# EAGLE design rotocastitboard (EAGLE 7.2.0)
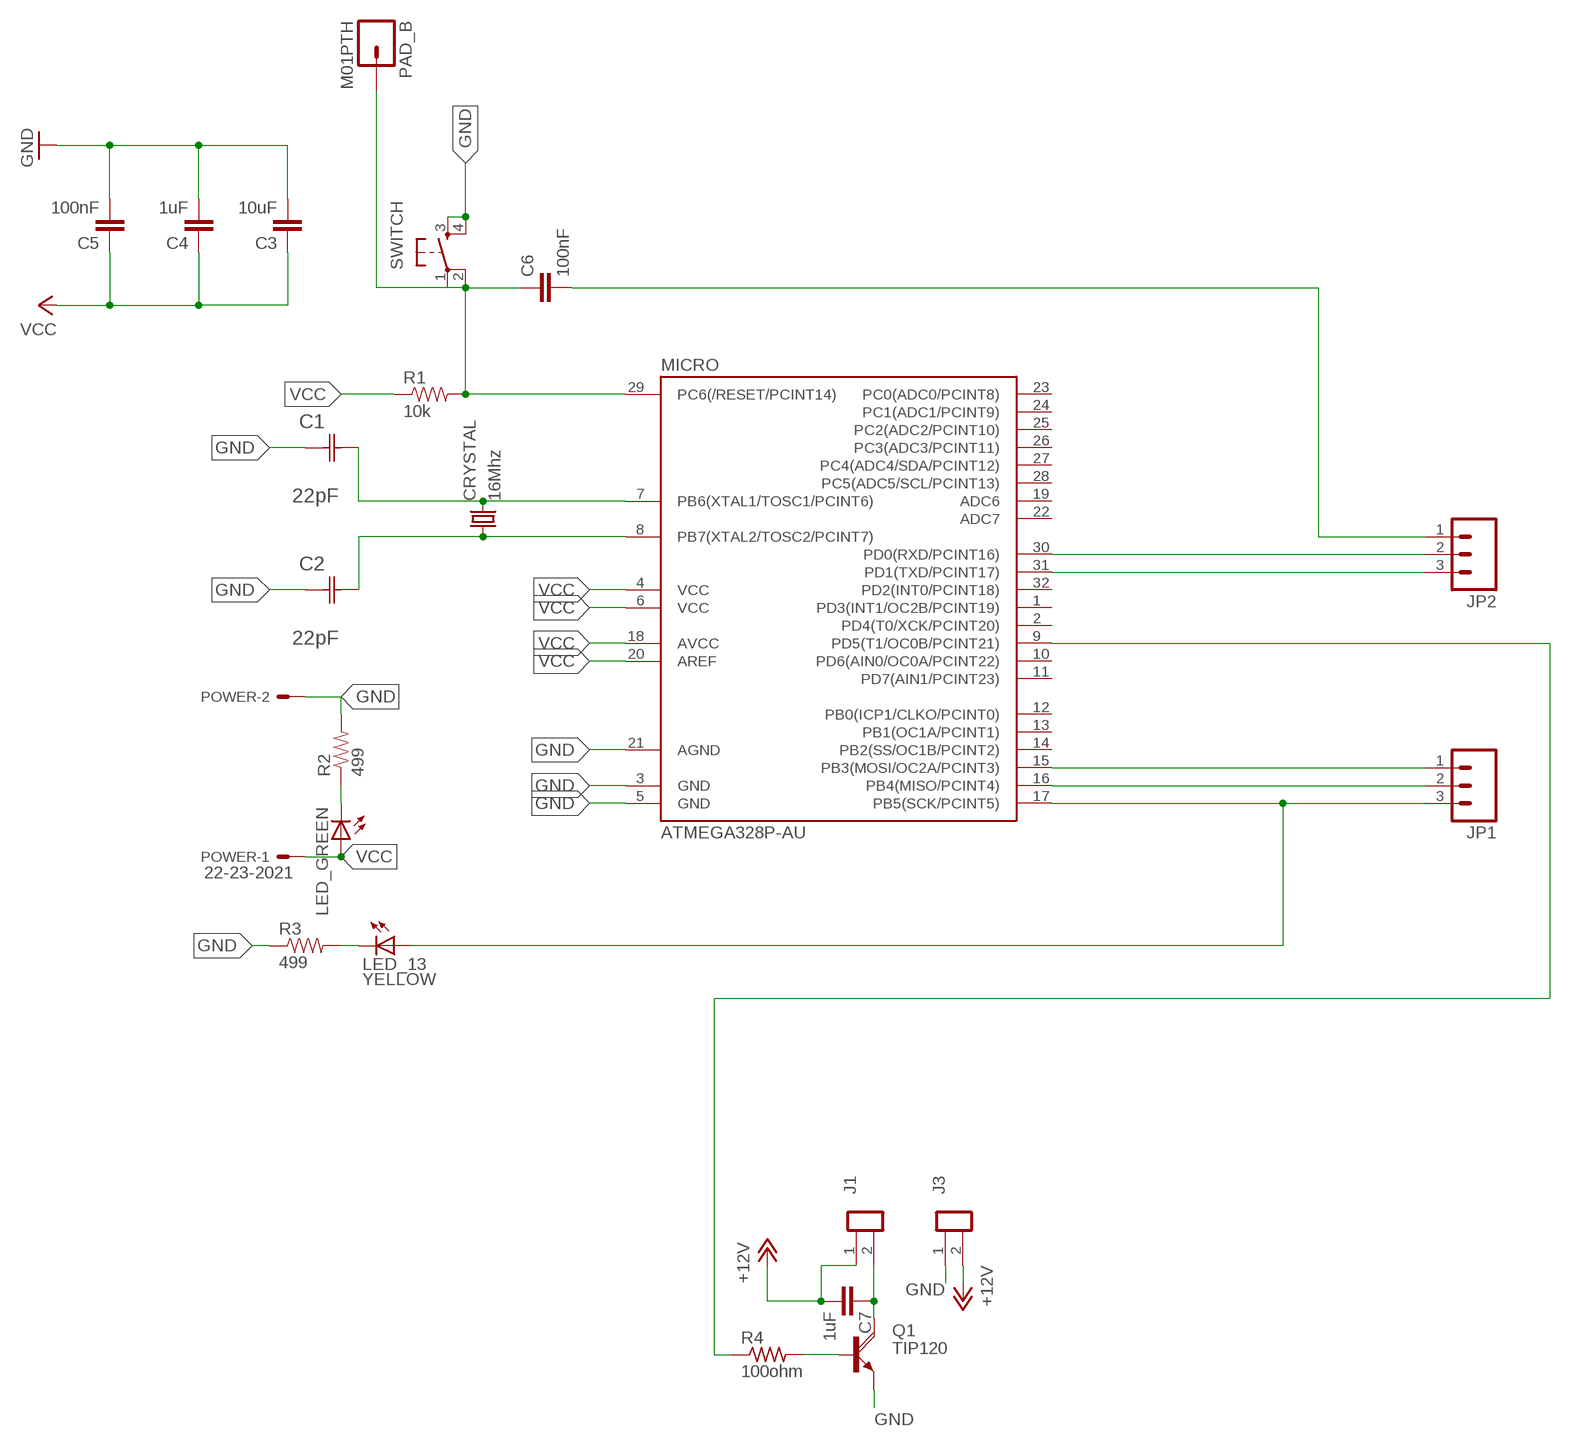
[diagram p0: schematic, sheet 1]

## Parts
C1  22pF  0612ZC225MAT2A  [CAPC3216X178N]
C2  22pF  0612ZC225MAT2A  [CAPC3216X178N]
C3  10uF  CAP1206  [1206]
C4  1uF  CAP1206  [1206]
C5  100nF  CAP1206  [1206]
C6  100nF  CAP1206  [1206]
C7  1uF  CAP1206  [1206]
CRYSTAL  16Mhz  CSM-7X-DU  [CSM-7X-DU]
J1  ED550-2  [ED550-2]
J3  ED550-2  [ED550-2]
JP1  M031X03_NO_SILK  [1X03_NO_SILK]
JP2  M031X03_NO_SILK  [1X03_NO_SILK]
LED_13  YELLOW  LED1206  [1206]
LED_GREEN  LED1206  [1206]
MICRO  ATMEGA328P-AU  ATMEGA48/88/168-AU  [TQFP32-08]
PAD_B  M01PTH  [1X01]
POWER  22-23-2021  [22-23-2021]
Q1  TIP120  [TO220AH]
R1  10k  RESISTOR1206  [1206]
R2  499  RESISTOR1206  [1206]
R3  499  RESISTOR1206  [1206]
R4  100ohm  RESISTOR1206  [1206]
SWITCH  6MM_SWITCH6MM_SWITCH  [6MM_SWITCH]

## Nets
+12V: C7.2 J1.1 J3.2
GND: C1.1(C1) C2.1(C1) C3.2 C4.2 C5.2 J3.1 MICRO.3(GND) MICRO.5(GND) MICRO.21(AGND) POWER.2 Q1.E R2.2 R3.1 SWITCH.3(S) SWITCH.4(S1)
N$1: C6.2 JP2.1
N$2: C1.2(C2) CRYSTAL.2 MICRO.7(PB6(XTAL1/TOSC1/PCINT6))
N$3: Q1.B R4.2
N$4: C7.1 J1.2 Q1.C
N$9: C2.2(C2) CRYSTAL.1 MICRO.8(PB7(XTAL2/TOSC2/PCINT7))
N$10: JP1.1 MICRO.15(PB3(MOSI/OC2A/PCINT3))
N$11: JP1.2 MICRO.16(PB4(MISO/PCINT4))
N$12: JP1.3 LED_13.1(A) MICRO.17(PB5(SCK/PCINT5))
N$20: JP2.2 MICRO.30(PD0(RXD/PCINT16))
N$21: JP2.3 MICRO.31(PD1(TXD/PCINT17))
N$26: LED_GREEN.2(C) R2.1
N$27: LED_13.2(C) R3.2
N$28: C6.1 MICRO.29(PC6(/RESET/PCINT14)) PAD_B.1 R1.2 SWITCH.1(P) SWITCH.2(P1)
N$34: MICRO.9(PD5(T1/OC0B/PCINT21)) R4.1
VCC: C3.1 C4.1 C5.1 LED_GREEN.1(A) MICRO.4(VCC) MICRO.6(VCC) MICRO.18(AVCC) MICRO.20(AREF) POWER.1 R1.1
Unconnected: MICRO.1(PD3(INT1/OC2B/PCINT19)) MICRO.2(PD4(T0/XCK/PCINT20)) MICRO.10(PD6(AIN0/OC0A/PCINT22)) MICRO.11(PD7(AIN1/PCINT23)) MICRO.12(PB0(ICP1/CLKO/PCINT0)) MICRO.13(PB1(OC1A/PCINT1)) MICRO.14(PB2(SS/OC1B/PCINT2)) MICRO.19(ADC6) MICRO.22(ADC7) MICRO.23(PC0(ADC0/PCINT8)) MICRO.24(PC1(ADC1/PCINT9)) MICRO.25(PC2(ADC2/PCINT10)) MICRO.26(PC3(ADC3/PCINT11)) MICRO.27(PC4(ADC4/SDA/PCINT12)) MICRO.28(PC5(ADC5/SCL/PCINT13)) MICRO.32(PD2(INT0/PCINT18))

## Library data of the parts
C1 C2 = AVX_By_element14_Batch_1:0612ZC225MAT2A: Capacitor 1206; MPN: 0612ZC225MAT2A; OC_FARNELL: -; OC_NEWARK: 12N3209; SUPPLIER: AVX; TOLERANCE: ±20%; VALUE: 2.2µF; VOLTAGERATING: 10V
C3-C7 = 01_SparkFun:CAP: Capacitor
CRYSTAL = 01_FAB_Hello:CSM-7X-DU: SMD CRYSTAL; OC_FARNELL: unknown; OC_NEWARK: unknown
J1 J3 = ads:ED550-2
JP1 JP2 = 01_SparkFun:M03: Header 3 Standard 3-pin 0.1" header. Use with straight break away headers (SKU : PRT-00116), right angle break away headers (PRT-00553), swiss pins (PRT-00743), machine pins (PRT-00117), and female headers (PRT-00115). Molex polarized connector foot print use with SKU : PRT-08232 with associated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
LED_13 LED_GREEN = 01_FAB_Hello:LED
MICRO = atmega8:ATMEGA48/88/168
PAD_B = 01_SparkFun:M01: Header 1
POWER = con-molex:22-23-2021: .100" (2.54mm) Center Header - 2 Pin; MF: MOLEX; MPN: 22-23-2021; OC_FARNELL: 1462926; OC_NEWARK: 25C3832
Q1 = transistor-power:TIP120: NPN DARLINGTON TRANSISTOR
R1-R3 = 01_SparkFun:RESISTOR: Resistor
R4 = 01_ng:RESISTOR
SWITCH = 01_FAB_Hello:6MM_SWITCH: OMRON SWITCH

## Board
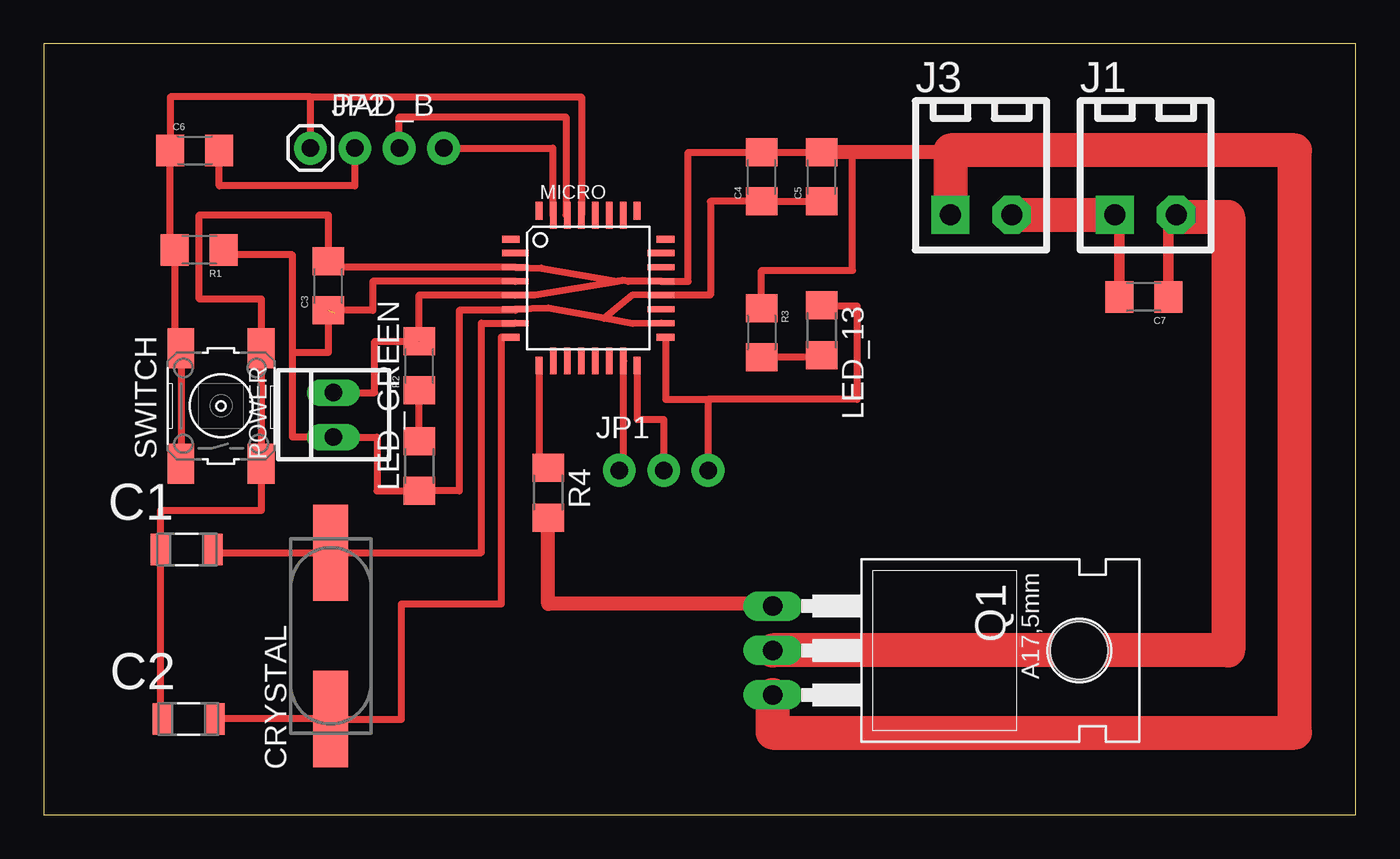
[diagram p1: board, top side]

Size 74.98 x 44.06 mm. Coordinates in mm from the lower left corner, seen from the top.
Outline: 0,0 74.98,0 74.98,44.06 0,44.06 0,0
Copper layers (1*16): Top 0.035mm / dielectric 1.5mm / Bottom 0.035mm
Design rules "default": minimum track width 10mil, minimum drill 24mil, track to track 8mil, track to pad 8mil, pad to pad 8mil, via to via 8mil, smd to smd 8mil, copper to edge 40mil, drill to drill 8mil, minimum pad ring 10mil, minimum via ring 8mil, stop-mask expansion 4mil, vias tented up to drill 0mil, thermal gap 10mil

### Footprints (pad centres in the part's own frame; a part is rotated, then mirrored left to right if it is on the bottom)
CAPC3216X178N = smd 1.118 x 1.803: 1 -1.499,0; 2 1.499,0
1206 = smd 1.6 x 1.8: 1 -1.4,0; 2 1.4,0
CSM-7X-DU = smd 5.5 x 2: 1 -4.75,0; 2 4.75,0
ED550-2 = drill 1.2 pad 2.184 square: 1 0,0 | drill 1.2 pad 2.184 octagon: 2 3.5,0
1X03_NO_SILK = drill 1.016 pad 1.88: 1 0,0; 2 2.54,0; 3 5.08,0
1206' = smd 1.6 x 1.803: 1 -1.422,0; 2 1.422,0
TQFP32-08 = smd 1.016 x 0.406: 1 -4.42,2.8; 8 -4.42,-2.8; 17 4.42,-2.8; 24 4.42,2.8 | smd 1.524 x 0.356: 2 -4.166,2; 3 -4.166,1.2; 4 -4.166,0.4; 5 -4.166,-0.4; 6 -4.166,-1.2; 7 -4.166,-2; 18 4.166,-2; 19 4.166,-1.2; 20 4.166,-0.4; 21 4.166,0.4; 22 4.166,1.2; 23 4.166,2 | smd 0.406 x 1.016: 9 -2.8,-4.42; 16 2.8,-4.42; 25 2.8,4.42; 32 -2.8,4.42 | smd 0.356 x 1.524: 10 -2,-4.166; 11 -1.2,-4.166; 12 -0.4,-4.166; 13 0.4,-4.166; 14 1.2,-4.166; 15 2,-4.166; 26 2,4.166; 27 1.2,4.166; 28 0.4,4.166; 29 -0.4,4.166; 30 -1.2,4.166; 31 -2,4.166
1X01 = drill 1.016 pad 1.88: 1 0,0
22-23-2021 = drill 1 long: 1 -1.27,0; 2 1.27,0
TO220AH = drill 1.118 long: B -2.54,-6.35; C 0,-6.35; E 2.54,-6.35 | hole 3.302: 0,11.176
6MM_SWITCH = smd 2.286 x 1.524: 1 -3.302,2.286; 2 3.302,2.286; 3 -3.302,-2.286; 4 3.302,-2.286

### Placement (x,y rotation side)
C1  8.18,15.16 0 top
C2  8.28,5.49 0 top
C3  16.26,30.23 90 top
C4  41.02,36.45 90 top
C5  44.45,36.45 90 top
C6  8.64,37.97 0 top
C7  62.86,29.59 180 top
CRYSTAL  16.41,10.24 90 top
J1  61.21,34.29 0 top
J3  51.82,34.29 0 top
JP1  32.89,19.69 0 top
JP2  17.78,38.1 0 top
LED_13  YELLOW  [1206']  44.45,27.69 270 top
LED_GREEN  [1206']  21.46,19.94 90 top
MICRO  31.11,30.1 0 top
PAD_B  15.24,38.1 0 top
POWER  16.56,22.86 90 top
Q1  48.01,9.4 270 top
R1  8.89,32.28 180 top
R2  21.46,25.65 90 top
R3  41.02,27.56 270 top
R4  100ohm  [1206']  28.83,18.41 270 top
SWITCH  10.13,23.37 90 top

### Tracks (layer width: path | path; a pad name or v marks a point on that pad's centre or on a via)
+12V
  Top 0.61: C7.2 61.47,34.29 J1.1
  Top 1.93: J3.2 J1.1
GND  (1 unrouted)
  Top 0.305: C2.1 6.68,5.49 | C1.1 6.6,15.16
  Top 0.406: POWER.2 18.92,24.13 18.92,27.05 R2.2 21.46,29.72 28.07,29.72 | 28.07,29.72 32.81,30.5 | 32.81,30.5 33.05,30.54 33.4,30.48 MICRO.21 35.28,30.48 36.83,30.48 36.83,37.85 C4.2 C5.2 46.23,37.85 46.23,31.12 41.02,31.12 R3.1 | 32.81,30.5 28.45,31.24 MICRO.3 16.58,31.3 arc-90 C3.2 16.26,34.29 8.89,34.29 8.89,29.46 12.45,29.46 12.45,26.67 SWITCH.4 SWITCH.3 12.45,20.07 12.45,17.4 6.68,17.4 C1.1 6.68,5.49 | MICRO.5 28.07,29.72
  Top 0.813: 51.82,37.97 51.82,37.85 C5.2
  Top 1.93: Q1.E 41.66,4.7 71.5,4.7 71.5,37.97 51.82,37.97 J3.1
N$1
  Top 0.406: JP2.1 17.78,35.94 10.03,35.94 C6.2
N$2
  Top 0.305: 9.68,14.99 | 9.68,14.99 C1.2
  Top 0.406: CRYSTAL.2 | CRYSTAL.2 25.02,14.99 25.02,28.1 MICRO.7 | 9.68,14.99 CRYSTAL.2
N$3
  Top 0.813: Q1.B 41.66,12.06 28.83,12.06 R4.2
N$4
  Top 0.61: C7.1 64.27,34.29 J1.2
  Top 1.93: J1.2 64.71,34.16 67.69,34.16 67.69,9.4 Q1.C
N$9
  Top 0.305: 9.78,5.46 C2.2 | C2.2
  Top 0.406: C2.2 CRYSTAL.1 16.41,5.46 20.45,5.46 20.45,12.06 26.16,12.06 26.16,27.3 MICRO.8
N$10
  Top 0.406: JP1.1 32.89,20.45 33.15,20.45 33.15,25.93 MICRO.15
N$11
  Top 0.406: MICRO.16 33.92,22.61 35.43,22.61 JP1.2
N$12
  Top 0.406: MICRO.17 35.53,23.75 37.97,23.75 | 37.97,23.75 JP1.3 | LED_13.1 44.45,29.08 46.48,29.08 46.48,23.75 37.97,23.75
N$20
  Top 0.406: JP2.2 20.32,39.88 29.85,39.88 29.85,34.27 MICRO.30
N$21
  Top 0.406: JP2.3 29.08,38.1 29.08,34.27 MICRO.31
N$26
  Top 0.406: LED_GREEN.2 R2.1
N$27
  Top 0.406: LED_13.2 44.45,26.16 R3.2
N$28
  Top 0.305: SWITCH.2 8.25,26.67
  Top 0.406: 7.75,20.07 SWITCH.1 SWITCH.2 7.49,26.67 R1.2 7.24,32.28 C6.1 7.24,41.02 15.24,41.02 | 15.24,41.02 30.73,41.02 30.73,34.27 MICRO.29 | PAD_B.1 15.24,41.02
N$34
  Top 0.406: MICRO.9 28.32,19.84 R4.1
VCC  (1 unrouted)
  Top 0.305: 16.64,28.7 16.64,28.58
  Top 0.406: 14.22,26.42 14.22,21.59 POWER.1 19.05,21.59 19.05,18.52 LED_GREEN.1 23.75,18.52 23.75,28.83 26.95,28.83 MICRO.6 28.83,28.96 32.02,28.37 | 14.22,26.42 14.22,32 10.29,32 R1.1 | 14.22,26.42 16.26,26.42 C3.1 18.8,28.83 18.8,30.48 26.95,30.48 MICRO.4 | MICRO.18 33.66,28.07 32.02,28.37 | 32.02,28.37 33.66,29.72 MICRO.20 38.1,29.7 38.1,35.05 C4.1 C5.1

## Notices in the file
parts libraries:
01_SparkFun: Licensing: CC v3.0 Share-Alike You are welcome to use this library for commercial purposes.
